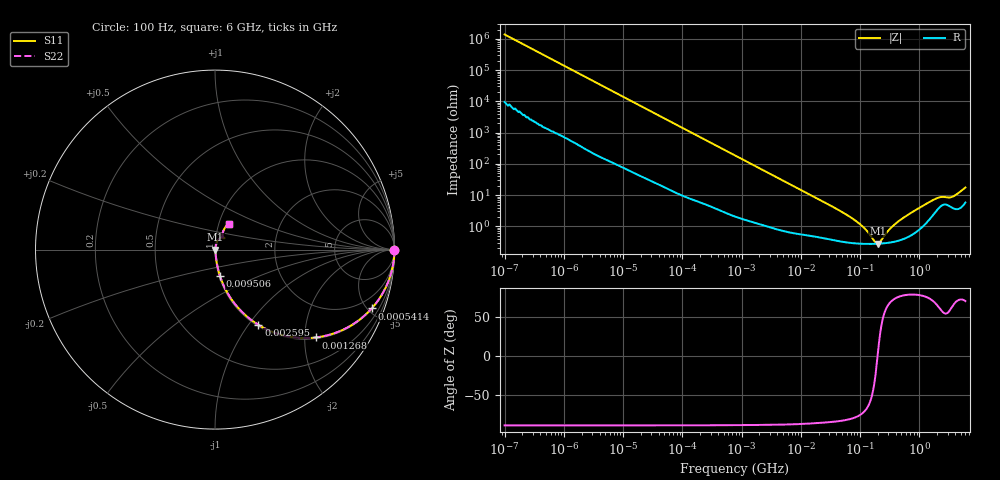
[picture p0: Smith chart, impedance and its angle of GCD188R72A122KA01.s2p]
!Murata Part Number: GCD188R72A122KA01
!These Parameters are Measured in Series Mode Connection
!Data Generated on Mar 13, 2026
!  o--ll--o
!Port1  Port2
!  o------o
!Operation Temp=25[degC], DC Bias Voltage=0[V]
!Freq. Start=100[Hz] Stop=6[GHz] 401[Steps]
# Hz S RI R 50
!Freq.(Hz) S11(Real) S11(Imag) S21(Real) S21(Imag) S12(Real) S12(Imag) S22(Real) S22(Imag)
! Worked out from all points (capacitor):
!   401 points, 100 Hz to 6 GHz, reference 50 ohm
!   read as one part in series: C = 1.14 nF near 109 Hz
!   lowest |Z| = 278 mohm at 199.7 MHz (marker M1)
!   series resonance near 197.7 MHz, so ESL is about 570 pH
!   S11 on the Smith chart (normalised r, x): 100 Hz: open; 541.4 kHz: 1.05, -5.30; 1.268 MHz: 1.03, -2.27; 2.595 MHz: 1.02, -1.12; 9.506 MHz: 1.01, -0.31; 6 GHz: 1.12, +0.33
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100  1 -7.2e-05  5e-07 7.2e-05  5e-07 7.2e-05  1 -7.2e-05
150  1 -0.000107  7e-07 0.000107  7e-07 0.000107  1 -0.000107
2008  1 -0.00143  9.1e-06 0.00143  9.1e-06 0.00143  1 -0.00143
40335  0.999 -0.0284  0.000983 0.0284  0.000983 0.0284  0.999 -0.0284
176758  0.9839 -0.1218  0.0161 0.1218  0.0161 0.1218  0.9839 -0.1218
541393  0.8729 -0.3281  0.1271 0.3281  0.1271 0.3281  0.8729 -0.3281
774597  0.7724 -0.4138  0.2276 0.4138  0.2276 0.4138  0.7724 -0.4138
1267578  0.5631 -0.4894  0.4369 0.4894  0.4369 0.4894  0.5631 -0.4894
2594782  0.2418 -0.4192  0.7582 0.4192  0.7582 0.4192  0.2418 -0.4192
4643984  0.0949 -0.2816  0.9051 0.2816  0.9051 0.2816  0.0949 -0.2816
9506416  0.0283 -0.1486  0.9717 0.1486  0.9717 0.1486  0.0283 -0.1486
1.555665e7  0.0135 -0.0926  0.9865 0.0926  0.9865 0.0926  0.0135 -0.0926
8.154455e7  0.00309 -0.0154  0.9969 0.0154  0.9969 0.0154  0.00309 -0.0154
1.220122e8  0.0028 -0.00772  0.9972 0.00772  0.9972 0.00772  0.0028 -0.00772
1.825626e8  0.00275 -0.00123  0.9972 0.00123  0.9972 0.00123  0.00275 -0.00123
1.996653e8  0.00277 0.000154  0.9972 -0.000154  0.9972 -0.000154  0.00277 0.000154
3.124326e8  0.00305 0.00731  0.9969 -0.00731  0.9969 -0.00731  0.00305 0.00731
5.346885e8  0.0042 0.018  0.9958 -0.018  0.9958 -0.018  0.0042 0.018
1.497423e9  0.0199 0.0563  0.9801 -0.0563  0.9801 -0.0563  0.0199 0.0563
2.240541e9  0.0451 0.0686  0.9549 -0.0686  0.9549 -0.0686  0.0451 0.0686
3.505958e9  0.0439 0.0704  0.9561 -0.0704  0.9561 -0.0704  0.0439 0.0704
6e9  0.0773 0.1441  0.9227 -0.1441  0.9227 -0.1441  0.0773 0.1441
